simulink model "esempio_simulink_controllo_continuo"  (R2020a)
settings: Solver=VariableStepAuto  StartTime=0.0  StopTime=250  RelTol=1e-3
undefined symbols (not defined in the file or in its folder): denGs, denRs, numGs, numRs

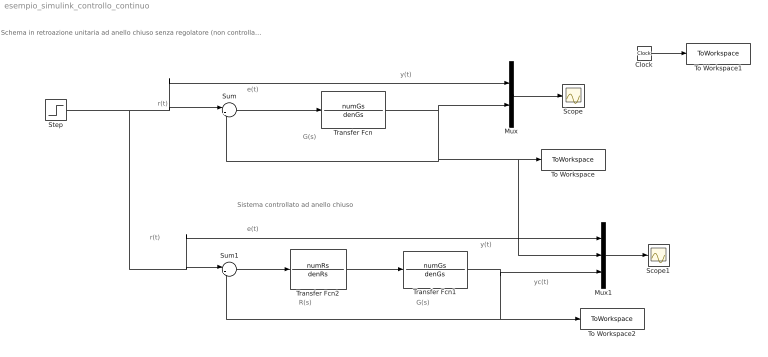
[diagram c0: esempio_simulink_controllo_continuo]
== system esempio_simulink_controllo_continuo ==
  note: Sistema controllato ad anello chiuso
  note: yc(t)
  note: R(s)
  note: e(t)
  note: y(t)
  note: r(t)
  note: Schema in retroazione unitaria ad anello chiuso senza regolatore (non controllato)
  note: G(s)
  note: y(t)
  note: r(t)
  note: e(t)
  note: G(s)
  Clock : Clock
  Mux : Mux  Inputs=2
  Mux1 : Mux  Inputs=3
  Scope : Scope
  Scope1 : Scope
  Step : Step  Time=0  SampleTime=0
  Sum : Sum  Inputs=|+-
  Sum1 : Sum  Inputs=|+-
  To Workspace : ToWorkspace  VariableName=ync  SampleTime=-1
  To Workspace1 : ToWorkspace  VariableName=tsim  SampleTime=-1
  To Workspace2 : ToWorkspace  VariableName=yc  SampleTime=-1
  Transfer Fcn : TransferFcn  Numerator=numGs  Denominator=denGs
  Transfer Fcn1 : TransferFcn  Numerator=numGs  Denominator=denGs
  Transfer Fcn2 : TransferFcn  Numerator=numRs  Denominator=denRs
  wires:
  Transfer Fcn/1 -> Mux/2, Sum/2, Mux1/2, To Workspace/1
  Step/1 -> Mux1/1, Sum1/1, Mux/1, Sum/1
  Sum/1 -> Transfer Fcn/1
  Mux/1 -> Scope/1
  Clock/1 -> To Workspace1/1
  Transfer Fcn1/1 -> Mux1/3, Sum1/2, To Workspace2/1
  Mux1/1 -> Scope1/1
  Sum1/1 -> Transfer Fcn2/1
  Transfer Fcn2/1 -> Transfer Fcn1/1
